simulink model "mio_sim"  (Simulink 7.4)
settings: Solver=ode45  StartTime=0.0  StopTime=3000  RelTol=1e-3
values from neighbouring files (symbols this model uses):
  dir = [V(2,1);V(2,2)]    [mio.m]
  F = [f11 0 f13 0; 0 f22 0 f24; 0 0 f33 0; 0 0 0 f44]    [mio.m]
  F_ = [f11_ 0 f13_ 0; 0 f22_ 0 f24_; 0 0 f33_ 0; 0 0 0 f44_]    [mio.m]
  G = [g11 0; 0 g22; 0 g32; g41 0]    [mio.m]
  G_ = [g11_ 0; 0 g22_; 0 g32_; g41_ 0]    [mio.m]
  H = H_    [mio.m]
  h1e = ((sqrt(2*g*h3e)*a3+gamma1*k1*v1)/(sqrt(2*g)*a1))^2    [mio.m]
  h2e = ((sqrt(2*g*h4e)*a4+gamma2*k2*v2)/(sqrt(2*g)*a2))^2    [mio.m]
  H_ = [kc 0 0 0; 0 kc 0 0]    [mio.m]
  kc = 0.5    [mio.m]
  ki1 = 0.09    [mio.m]
  ki2 = -0.001    [mio.m]
  kp1 = 4.5    [mio.m]
  kp2 = -0.1    [mio.m]
libraries: cstblocks x2

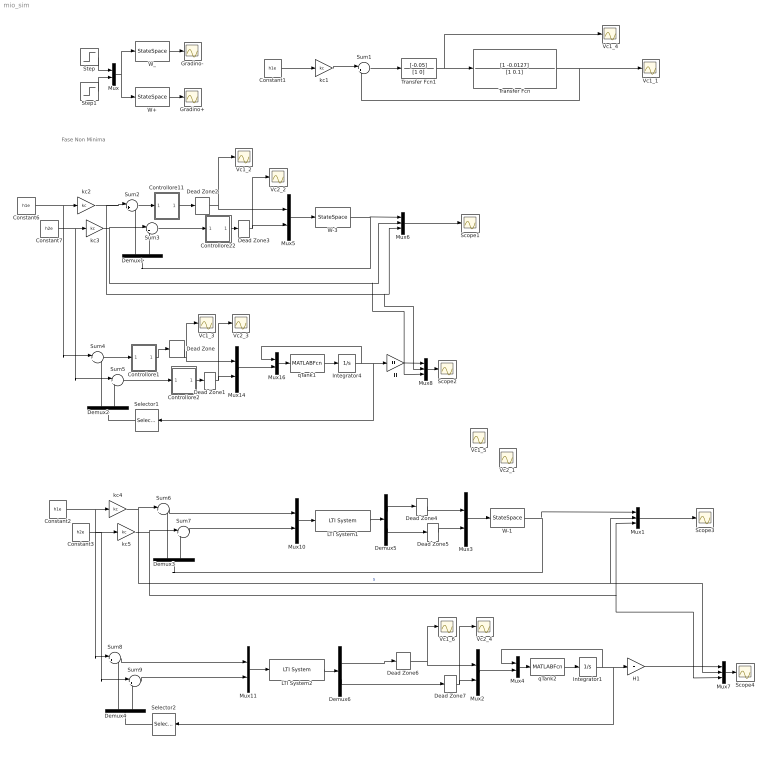
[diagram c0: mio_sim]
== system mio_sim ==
  note: Fase Non Minima
  Constant1 : Constant  Value=h1e  OutDataType=sfix(16)  OutScaling=2^0
  Constant2 : Constant  Value=h1e  OutDataType=sfix(16)  OutScaling=2^0
  Constant3 : Constant  Value=h2e  OutDataType=sfix(16)  OutScaling=2^0
  Constant6 : Constant  Value=h1e  OutDataType=sfix(16)  OutScaling=2^0
  Constant7 : Constant  Value=h2e  OutDataType=sfix(16)  OutScaling=2^0
  Controllore1 : Subsystem
  Controllore11 : Subsystem
  Controllore2 : Subsystem
  Controllore22 : Subsystem
  Dead Zone{,1..7} (8 alike) : DeadZone  LowerValue=-100000  UpperValue=0
  Demux{1..6} (6 alike) : Demux  Outputs=2
  Gradino+ : Scope
  Gradino- : Scope
  H : Gain  Gain=H  Multiplication=Matrix(K*u)  ParameterDataType=sfix(16)  ParameterScaling=2^0  OutDataType=sfix(16)  OutScaling=2^0
  H1 : Gain  Gain=H  Multiplication=Matrix(K*u)  ParameterDataType=sfix(16)  ParameterScaling=2^0  OutDataType=sfix(16)  OutScaling=2^0
  Integrator1 : Integrator
  Integrator4 : Integrator
  LTI System1 : cstblocks/LTI System  SystemSampleTime=-1  sys=Cont_dec_simp  IC=[]
  LTI System2 : cstblocks/LTI System  SystemSampleTime=-1  sys=Cont_dec_simp  IC=[]
  Mux{,2..5,10..11,14,16} (9 alike) : Mux  Inputs=2
  Mux{1,6..8} (4 alike) : Mux  Inputs=3
  Scope{1..4} (4 alike) : Scope
  Selector1 : Selector  InputPortWidth=4  IndexOptions=Index vector (dialog)  Indices=[1 2]  OutputSizes=1
  Selector2 : Selector  InputPortWidth=4  IndexOptions=Index vector (dialog)  Indices=[1 2]  OutputSizes=1
  Step : Step  Time=0  After=dir(1)  SampleTime=0
  Step1 : Step  Time=0  After=dir(2)  SampleTime=0
  Sum{1..9} (9 alike) : Sum  Inputs=|+-  OutDataType=sfix(16)  OutScaling=2^0
  Transfer Fcn : TransferFcn  Numerator=[1 -0.0127]  Denominator=[1 0.1]
  Transfer Fcn1 : TransferFcn  Numerator=[-0.05]  Denominator=[1 0]
  Vc1_{1..6} (6 alike) : Scope
  Vc2_{1..4} (4 alike) : Scope
  W+ : StateSpace  A=F  B=G  C=H  D=zeros(2)
  W-1 : StateSpace  A=F  B=G  C=H  D=zeros(2)
  W-3 : StateSpace  A=F  B=G  C=H  D=zeros(2)
  W_ : StateSpace  A=F_  B=G_  C=H_  D=zeros(2)
  kc{1..5} (5 alike) : Gain  Gain=kc  ParameterDataType=sfix(16)  ParameterScaling=2^0  OutDataType=sfix(16)  OutScaling=2^0
  qTank1 : MATLABFcn  MATLABFcn=qTank  OutputDimensions=4
  qTank2 : MATLABFcn  MATLABFcn=qTank  OutputDimensions=4
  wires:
  W_/1 -> Gradino-/1
  W+/1 -> Gradino+/1
  Mux/1 -> W+/1, W_/1
  Step/1 -> Mux/1
  Step1/1 -> Mux/2
  Sum2/1 -> Controllore11/1(In1)
  Constant6/1 -> kc2/1, Sum4/1
  Sum3/1 -> Controllore22/1(In1)
  Constant7/1 -> kc3/1, Sum5/1
  Demux1/2 -> Sum3/2
  Demux1/1 -> Sum2/2
  Mux5/1 -> W-3/1
  Mux6/1 -> Scope1/1
  Controllore11/1(Out1) -> Dead Zone2/1
  Controllore22/1(Out1) -> Dead Zone3/1
  qTank1/1 -> Integrator4/1
  Sum4/1 -> Controllore1/1(In1)
  Sum5/1 -> Controllore2/1(In1)
  Demux2/2 -> Sum5/2
  Demux2/1 -> Sum4/2
  Controllore1/1(Out1) -> Dead Zone/1
  Controllore2/1(Out1) -> Dead Zone1/1
  Integrator4/1 -> H/1, Selector1/1, Mux16/1
  Mux16/1 -> qTank1/1
  Mux14/1 -> Mux16/2
  W-3/1 -> Mux6/1, Demux1/1
  Selector1/1 -> Demux2/1
  Mux8/1 -> Scope2/1
  H/1 -> Mux8/1
  kc2/1 -> Sum2/1, Mux6/3, Mux8/2
  kc3/1 -> Sum3/1, Mux6/2, Mux8/3
  Dead Zone/1 -> Mux14/1, Vc1_3/1
  Dead Zone1/1 -> Vc2_3/1, Mux14/2
  Dead Zone2/1 -> Vc1_2/1, Mux5/1
  Dead Zone3/1 -> Vc2_2/1, Mux5/2
  Constant1/1 -> kc1/1
  Sum1/1 -> Transfer Fcn1/1
  kc1/1 -> Sum1/1
  Transfer Fcn/1 -> Sum1/2, Vc1_1/1
  Transfer Fcn1/1 -> Transfer Fcn/1, Vc1_4/1
  Constant2/1 -> kc4/1, Sum8/1
  Constant3/1 -> kc5/1, Sum9/1
  Demux3/2 -> Sum7/2
  Demux3/1 -> Sum6/2
  Mux3/1 -> W-1/1
  W-1/1 -> Demux3/1, Mux1/1
  kc4/1 -> Sum6/1, Mux1/2, Mux7/2  "s"
  kc5/1 -> Sum7/1, Mux1/3, Mux7/3
  Mux10/1 -> LTI System1/1
  LTI System1/1 -> Demux5/1
  Sum7/1 -> Mux10/2
  Sum6/1 -> Mux10/1
  Demux5/1 -> Dead Zone4/1
  Dead Zone4/1 -> Mux3/1
  Dead Zone5/1 -> Mux3/2
  Demux5/2 -> Dead Zone5/1
  Mux1/1 -> Scope3/1
  qTank2/1 -> Integrator1/1
  Demux4/2 -> Sum9/2
  Demux4/1 -> Sum8/2
  Integrator1/1 -> H1/1, Selector2/1, Mux4/1
  Mux4/1 -> qTank2/1
  Mux2/1 -> Mux4/2
  Selector2/1 -> Demux4/1
  Mux7/1 -> Scope4/1
  H1/1 -> Mux7/1
  Dead Zone6/1 -> Mux2/1, Vc1_6/1
  Dead Zone7/1 -> Vc2_4/1, Mux2/2
  Mux11/1 -> LTI System2/1
  LTI System2/1 -> Demux6/1
  Sum9/1 -> Mux11/2
  Sum8/1 -> Mux11/1
  Demux6/1 -> Dead Zone6/1
  Demux6/2 -> Dead Zone7/1

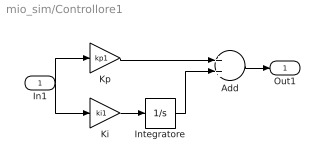
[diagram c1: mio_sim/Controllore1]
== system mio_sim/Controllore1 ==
  In1 : Inport
  Add : Sum  OutDataType=sfix(16)  OutScaling=2^-10
  Integratore : Integrator
  Ki : Gain  Gain=ki1  ParameterDataType=sfix(16)  ParameterScaling=2^0  OutDataType=sfix(16)  OutScaling=2^0
  Kp : Gain  Gain=kp1  ParameterDataType=sfix(16)  ParameterScaling=2^0  OutDataType=sfix(16)  OutScaling=2^0
  Out1 : Outport
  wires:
  Add/1 -> Out1/1
  In1/1 -> Ki/1, Kp/1
  Integratore/1 -> Add/2
  Kp/1 -> Add/1
  Ki/1 -> Integratore/1

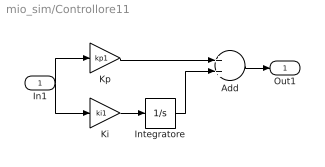
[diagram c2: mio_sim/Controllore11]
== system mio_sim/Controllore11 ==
  In1 : Inport
  Add : Sum  OutDataType=sfix(16)  OutScaling=2^-10
  Integratore : Integrator
  Ki : Gain  Gain=ki1  ParameterDataType=sfix(16)  ParameterScaling=2^0  OutDataType=sfix(16)  OutScaling=2^0
  Kp : Gain  Gain=kp1  ParameterDataType=sfix(16)  ParameterScaling=2^0  OutDataType=sfix(16)  OutScaling=2^0
  Out1 : Outport
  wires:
  Add/1 -> Out1/1
  In1/1 -> Ki/1, Kp/1
  Integratore/1 -> Add/2
  Kp/1 -> Add/1
  Ki/1 -> Integratore/1

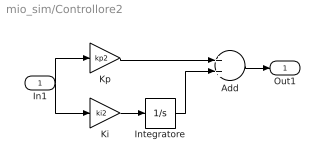
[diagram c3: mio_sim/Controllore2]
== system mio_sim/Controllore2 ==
  In1 : Inport
  Add : Sum  OutDataType=sfix(16)  OutScaling=2^-10
  Integratore : Integrator
  Ki : Gain  Gain=ki2  ParameterDataType=sfix(16)  ParameterScaling=2^0  OutDataType=sfix(16)  OutScaling=2^0
  Kp : Gain  Gain=kp2  ParameterDataType=sfix(16)  ParameterScaling=2^0  OutDataType=sfix(16)  OutScaling=2^0
  Out1 : Outport
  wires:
  Add/1 -> Out1/1
  In1/1 -> Ki/1, Kp/1
  Integratore/1 -> Add/2
  Kp/1 -> Add/1
  Ki/1 -> Integratore/1

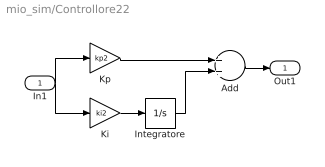
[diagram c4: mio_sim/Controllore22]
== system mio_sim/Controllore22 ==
  In1 : Inport
  Add : Sum  OutDataType=sfix(16)  OutScaling=2^-10
  Integratore : Integrator
  Ki : Gain  Gain=ki2  ParameterDataType=sfix(16)  ParameterScaling=2^0  OutDataType=sfix(16)  OutScaling=2^0
  Kp : Gain  Gain=kp2  ParameterDataType=sfix(16)  ParameterScaling=2^0  OutDataType=sfix(16)  OutScaling=2^0
  Out1 : Outport
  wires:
  Add/1 -> Out1/1
  In1/1 -> Ki/1, Kp/1
  Integratore/1 -> Add/2
  Kp/1 -> Add/1
  Ki/1 -> Integratore/1
